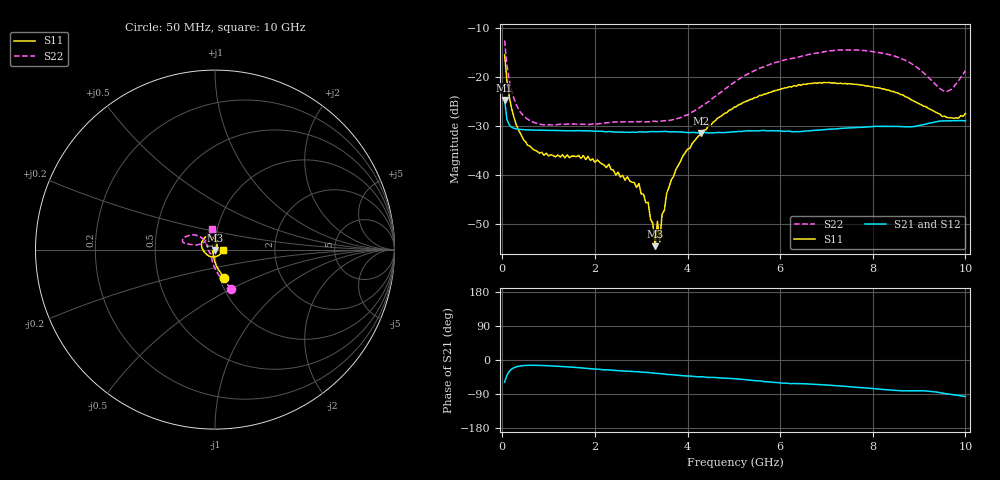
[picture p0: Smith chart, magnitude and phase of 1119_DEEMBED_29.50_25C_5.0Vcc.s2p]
!Hittite Microwave Corp.
!Digital Attenuator/PhaseShifter Rev 1.4.0
!Filename: C:\DATA\DATA\1119_DEEMBED_29.50_25C_5.0Vcc.s2p
!VNA ID: Agilent Technologies,N5224A,MY51441122,A.10.45.03
!Device type:
!2 Port Calibration.
!Temp(C): 25
!Lot Number:
!Serial Number:
!Operator:
!Misc:
!Attenuator:  29.500
# GHZ S DB R 50.0
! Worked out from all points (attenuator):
!   200 points, 50 MHz to 10 GHz, reference 50 ohm
!   highest |S21| = -24.68 dB at 50 MHz (marker M1); lowest = -31.5 dB at 4.3 GHz (marker M2)
!   lowest |S11| = -54.5 dB at 3.3 GHz (marker M3), VSWR 1.00, Z = 50.1 - j0.14 ohm
!   |S11| at or under -10 dB: start of sweep to end of sweep
!   |S22| runs from -29.8 to -12.6 dB; largest |S21 - S12| = 0.00015
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0.05  -15.48 -72.4  -24.68 -58.6  -24.70 -58.7  -12.56 -67.5
0.1  -20.78 -85.2  -28.69 -40.3  -28.69 -40.3  -17.51 -84.0
0.2  -26.39 -97.6  -30.26 -23.9  -30.26 -23.9  -22.78 -100.6
0.35  -30.85 -109.3  -30.69 -16.6  -30.69 -16.5  -26.56 -114.7
0.55  -33.97 -123.1  -30.82 -14.2  -30.81 -14.1  -28.65 -126.5
0.9  -36.00 -135.6  -30.90 -14.7  -30.90 -14.7  -29.76 -135.9
1.75  -36.04 -142.1  -31.00 -21.3  -31.00 -21.3  -29.67 -140.9
2.95  -41.78 -105.8  -31.22 -31.2  -31.23 -31.3  -29.14 -160.2
3.15  -45.61 -84.0  -31.21 -32.9  -31.21 -33.0  -29.14 -166.3
3.2  -49.03 -79.5  -31.17 -33.6  -31.17 -33.6  -29.14 -167.5
3.25  -49.90 -55.3  -31.15 -34.4  -31.16 -34.5  -29.02 -169.0
3.3  -54.55 -48.0  -31.17 -35.0  -31.18 -35.1  -29.07 -170.7
3.35  -49.47 -9.3  -31.19 -35.4  -31.20 -35.5  -29.11 -172.4
3.4  -53.69 8.3  -31.16 -35.7  -31.17 -35.7  -29.05 -173.8
3.45  -48.08 30.3  -31.17 -36.4  -31.17 -36.5  -28.98 -175.7
3.65  -40.99 49.0  -31.24 -38.6  -31.25 -38.7  -28.82 177.1
4.3  -31.67 66.8  -31.46 -44.2  -31.47 -44.3  -25.99 150.4
5.05  -26.10 83.6  -31.18 -49.8  -31.20 -49.8  -20.83 138.6
6.7  -21.32 124.1  -30.94 -64.0  -30.94 -63.9  -15.26 153.8
8.35  -22.71 172.5  -30.11 -78.9  -30.10 -78.9  -15.44 168.1
9.55  -28.01 -80.9  -28.96 -88.3  -28.97 -88.4  -22.88 138.1
10  -27.46 -5.4  -28.97 -96.4  -28.98 -96.4  -18.75 98.2
